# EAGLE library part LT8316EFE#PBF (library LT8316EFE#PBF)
Switching Controllers 600VIN Micropower, Isolated No-Opto Flyb Source: Datasheet
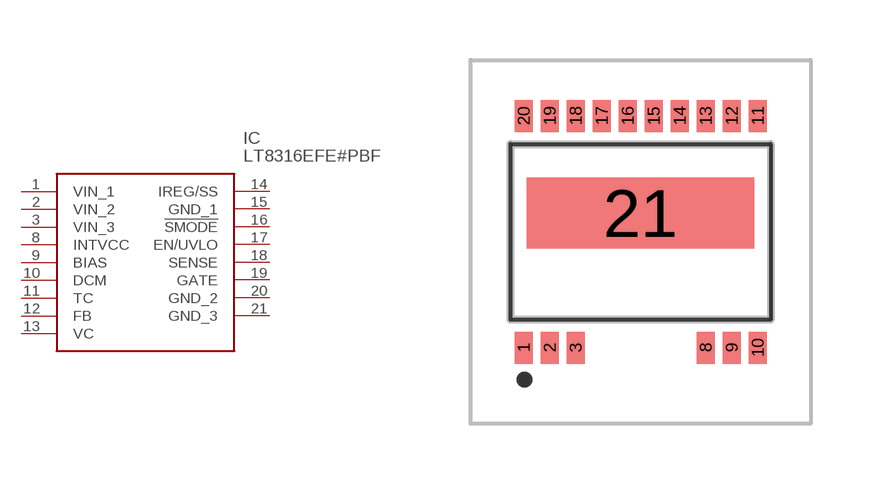
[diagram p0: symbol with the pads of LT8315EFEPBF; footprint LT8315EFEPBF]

Designator prefix IC

## LT8316EFE#PBF (Description: Switching Controllers 600VIN Micropower, Isolated No-Opto Flyb; Height: 1mm; Manufacturer_Name: Analog Devices; Manufacturer_Part_Number: LT8316EFE#PBF; Mouser_Part_Number: 584-LT8316EFE#PBF; Mouser_Price-Stock: https://www.mouser.co.uk/ProductDetail/Analog-Devices/LT8316EFEPBF?qs=0lSvoLzn4L9vCHQJkSIf7Q%3D%3D)  [LT8315EFEPBF]
1  VIN_1
2  VIN_2
3  VIN_3
8  INTVCC
9  BIAS
10  DCM
11  TC
12  FB
13  VC
14  IREG/SS
15  GND_1
16  !SMODE
17  EN/UVLO
18  SENSE
19  GATE
20  GND_2
21  GND_3

## Footprint LT8315EFEPBF (pad centres in mm)
FE Package Variation: FE20(16) 20-Lead Plastic TSSOP (4.4mm) (Reference LTC DWG # 05-08-1990 Rev &Oslash;)
smd 0.45 x 0.8: 1 -2.925,-2.45; 2 -2.275,-2.45; 3 -1.625,-2.45; 8 1.625,-2.45; 9 2.275,-2.45; 10 2.925,-2.45; 11 2.925,3.35; 12 2.275,3.35; 13 1.625,3.35; 14 0.975,3.35; 15 0.325,3.35; 16 -0.325,3.35; 17 -0.975,3.35; 18 -1.625,3.35; 19 -2.275,3.35; 20 -2.925,3.35
smd 5.68 x 1.78: 21 0,0.92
